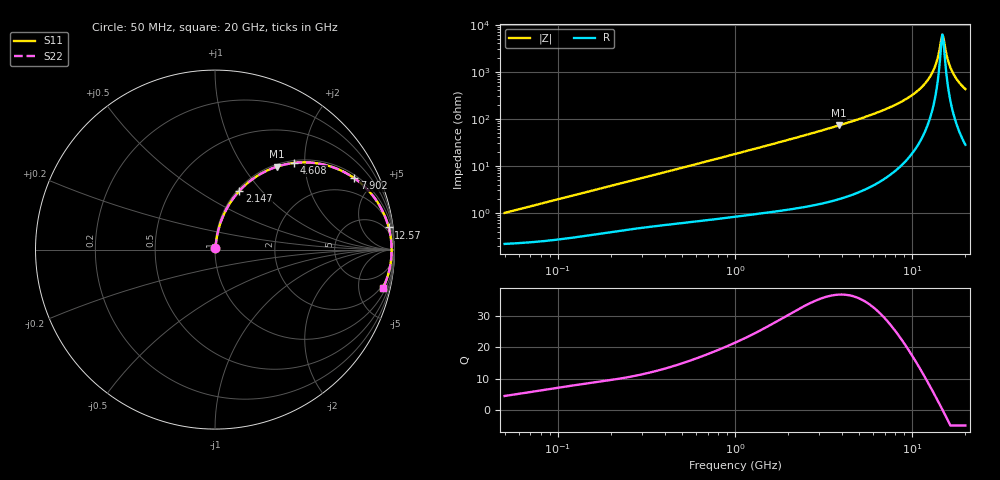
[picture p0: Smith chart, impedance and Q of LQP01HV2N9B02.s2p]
!Murata Part Number: LQP01HV2N9B02
!These Parameters are Measured in Series Mode Connection
!  o--[Z]--o
!Port1  Port2
!  o-------o
!Freq. Start=50[MHz] Stop=20[GHz], 401[Steps]
# Hz S RI R 50
!Freq.(Hz) S11(Real) S11(Imag) S21(Real) S21(Imag) S12(Real) S12(Imag) S22(Real) S22(Imag)
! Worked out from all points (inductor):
!   401 points, 50 MHz to 20 GHz, reference 50 ohm
!   read as one part in series: L = 3.09 nH near 51.52 MHz
!   highest Q = 36.9 at 3.85 GHz (marker M1), where L = 2.97 nH
!   self-resonance near 14.82 GHz
!   S11 on the Smith chart (normalised r, x): 50 MHz: 1.00, +0.02; 2.147 GHz: 1.02, +0.77; 4.608 GHz: 1.05, +1.77; 7.902 GHz: 1.15, +3.83; 12.57 GHz: 3, +15; 20 GHz: 1.56, -8.52
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5e7  0.00228 0.00971  0.9977 -0.00971  0.9977 -0.00971  0.00228 0.00971
1.364002e8  0.00383 0.0258  0.9962 -0.0258  0.9962 -0.0258  0.00383 0.0258
3.721004e8  0.00982 0.0668  0.9902 -0.0668  0.9902 -0.0668  0.00982 0.0668
1e9  0.0381 0.1697  0.9619 -0.1697  0.9619 -0.1697  0.0381 0.1697
2.146657e9  0.1361 0.3274  0.8639 -0.3274  0.8639 -0.3274  0.1361 0.3274
2.728004e9  0.2024 0.3875  0.7976 -0.3875  0.7976 -0.3875  0.2024 0.3875
3.850025e9  0.3448 0.462  0.6552 -0.462  0.6552 -0.462  0.3448 0.462
4.608136e9  0.4423 0.4831  0.5577 -0.4831  0.5577 -0.4831  0.4423 0.4831
7.442007e9  0.7414 0.4201  0.2586 -0.4201  0.2586 -0.4201  0.7414 0.4201
7.901521e9  0.777 0.3973  0.223 -0.3973  0.223 -0.3973  0.777 0.3973
1.050288e10  0.9163 0.2465  0.0837 -0.2465  0.0837 -0.2465  0.9163 0.2465
1.166392e10  0.9504 0.1766  0.0496 -0.1766  0.0496 -0.1766  0.9504 0.1766
1.257102e10  0.9678 0.1235  0.0322 -0.1235  0.0322 -0.1235  0.9678 0.1235
1.354865e10  0.979 0.0687  0.021 -0.0687  0.021 -0.0687  0.979 0.0687
1.460232e10  0.9839 0.0128  0.0161 -0.0128  0.0161 -0.0128  0.9839 0.0128
1.482269e10  0.9841 0.00154  0.0159 -0.00154  0.0159 -0.00154  0.9841 0.00154
1.504638e10  0.9841 -0.0097  0.0159 0.0097  0.0159 0.0097  0.9841 -0.0097
1.527346e10  0.9838 -0.0209  0.0162 0.0209  0.0162 0.0209  0.9838 -0.0209
1.597544e10  0.9813 -0.0545  0.0187 0.0545  0.0187 0.0545  0.9813 -0.0545
1.696185e10  0.9745 -0.0989  0.0255 0.0989  0.0255 0.0989  0.9745 -0.0989
1.828096e10  0.9602 -0.1532  0.0398 0.1532  0.0398 0.1532  0.9602 -0.1532
2e10  0.9352 -0.2154  0.0648 0.2154  0.0648 0.2154  0.9352 -0.2154
